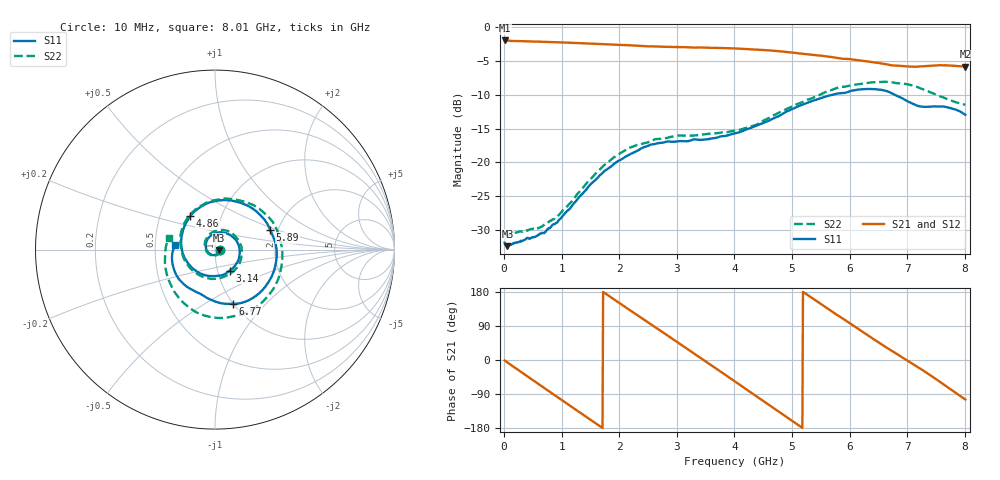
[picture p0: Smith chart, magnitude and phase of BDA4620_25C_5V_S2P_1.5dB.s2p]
!Agilent Technologies,E5071B,MY42404982,A.09.10
!Date: Wed May 06 08:58:23 2026
!Data & Calibration Information:
!Freq	S11:SOLT2(ON)	S21:SOLT2(ON)	S12:SOLT2(ON)	S22:SOLT2(ON)
# Hz S RI R 50
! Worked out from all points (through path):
!   801 points, 10 MHz to 8.01 GHz, reference 50 ohm
!   highest |S21| = -1.95 dB at 10 MHz (marker M1); lowest = -5.8 dB at 8.01 GHz (marker M2)
!   group delay of S21, straight-line fit = 286 ps
!   lowest |S11| = -32.4 dB at 60 MHz (marker M3), VSWR 1.05, Z = 52.4 - j0.332 ohm
!   |S11| at or under -10 dB: start of sweep to 5.701 GHz; 6.785 GHz to end of sweep
!   |S22| runs from -30.8 to -8.1 dB; largest |S21 - S12| = 0.0035
!   S11 on the Smith chart (normalised r, x): 10 MHz: 1.05, -0.00; 3.14 GHz: 1.15, -0.27; 4.86 GHz: 0.71, +0.28; 5.89 GHz: 1.81, +0.45; 6.77 GHz: 1.00, -0.67; 8.01 GHz: 0.63, +0.03
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1e7  0.0254 -0.00177  0.7984 -0.0168  0.7994 -0.0173  0.0304 -0.00199
6e7  0.0238 -0.00317  0.7899 -0.0915  0.7914 -0.093  0.0289 -0.00345
3.6e8  0.0201 -0.0176  0.6184 -0.488  0.6186 -0.4891  0.0233 -0.0204
7.3e8  -0.00546 -0.0306  0.1728 -0.7596  0.1726 -0.7607  -0.00543 -0.0348
1.03e9  -0.037 -0.017  -0.2454 -0.7307  -0.2464 -0.7317  -0.0401 -0.0197
1.35e9  -0.0517 0.0264  -0.6003 -0.469  -0.601 -0.4696  -0.0574 0.0272
1.64e9  -0.0299 0.0723  -0.7451 -0.1034  -0.7463 -0.1035  -0.0369 0.0785
1.93e9  0.0229 0.0963  -0.6881 0.2794  -0.6888 0.2804  0.0198 0.1087
2.32e9  0.1027 0.0669  -0.3377 0.6474  -0.3386 0.648  0.109 0.0796
2.68e9  0.1383 -0.0152  0.1142 0.7106  0.1152 0.7114  0.1491 -0.00106
3.14e9  0.0831 -0.117  0.5933 0.3946  0.5948 0.3936  0.1075 -0.116
3.57e9  -0.0221 -0.1472  0.6925 -0.1313  0.6933 -0.133  -0.00625 -0.1632
4.01e9  -0.1329 -0.096  0.3817 -0.5824  0.3814 -0.5837  -0.1354 -0.1068
4.43e9  -0.1883 0.0294  -0.1265 -0.6697  -0.1272 -0.6699  -0.1921 0.0309
4.86e9  -0.1384 0.1862  -0.5468 -0.3689  -0.5475 -0.3691  -0.1262 0.2081
5.35e9  0.0746 0.2753  -0.5985 0.179  -0.5993 0.1794  0.1076 0.279
5.89e9  0.307 0.1105  -0.1852 0.5541  -0.1846 0.5548  0.3503 0.0936
6.25e9  0.3339 -0.0994  0.1751 0.5346  0.1766 0.5353  0.364 -0.1243
6.68e9  0.1524 -0.2957  0.4612 0.2548  0.4633 0.2551  0.1964 -0.3423
6.77e9  0.0998 -0.3026  0.4872 0.1839  0.4894 0.1833  0.1397 -0.363
7.34e9  -0.1176 -0.2294  0.4281 -0.289  0.4297 -0.2902  -0.1925 -0.2787
8.01e9  -0.2238 0.0231  -0.1262 -0.4944  -0.1266 -0.4957  -0.2585 0.066
